(* Logix 5000 AddOnInstructionDefinition export; software revision 16.04 *)

ADD_ON_INSTRUCTION AMCI_ANG1E_Disable_Driver   (* revision 1.1, vendor AMCI *)
// Revision note:
// Version 1.1 added the slot_axis number and the input parameters can now be tags or discrete values.
VAR_INPUT
   slot_axis_number : INT; {required}
END_VAR
VAR_IN_OUT
   AMCI_ANG1E_output_data : INT[10]; {required}
END_VAR
VAR
   command_data_block : INT[10];
        [0]   // Command Bits MSW
        [1]   // Command Bits LSW
        [2]   // Upper Target Position
        [3]   // Lower Target Position
        [4]   // Upper Programmed Speed
        [5]   // Lower Programmed Speed
   index : INT;
END_VAR

ROUTINE Logic   (* ladder *)
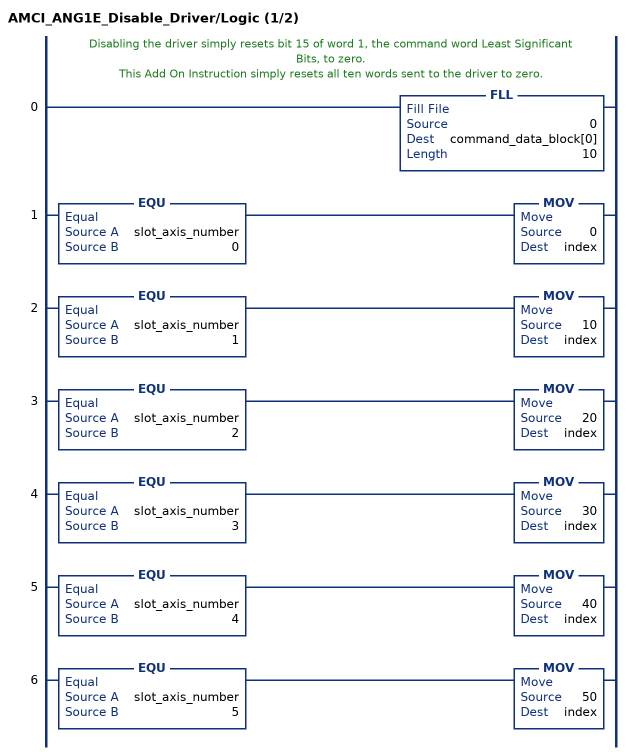
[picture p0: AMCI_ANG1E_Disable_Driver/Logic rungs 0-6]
   // Disabling the driver simply resets bit 15 of word 1, the command word Least Significant Bits, to zero.
   // This Add On Instruction simply resets all ten words sent to the driver to zero.
   0: FLL(0,command_data_block[0],10);
   1: EQU(slot_axis_number,0)MOV(0,index);
   2: EQU(slot_axis_number,1)MOV(10,index);
   3: EQU(slot_axis_number,2)MOV(20,index);
   4: EQU(slot_axis_number,3)MOV(30,index);
   5: EQU(slot_axis_number,4)MOV(40,index);
   6: EQU(slot_axis_number,5)MOV(50,index);
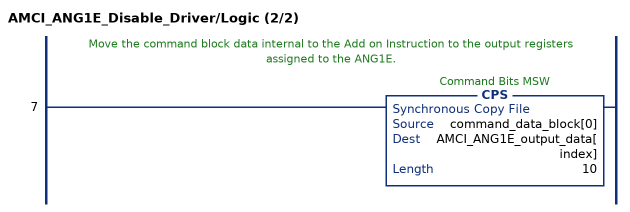
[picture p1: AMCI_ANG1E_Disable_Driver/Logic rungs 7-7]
   // Move the command block data internal to the Add on Instruction to the output registers assigned to the ANG1E.
   7: CPS(command_data_block[0],AMCI_ANG1E_output_data[index],10);
END_ROUTINE
END_ADD_ON_INSTRUCTION
